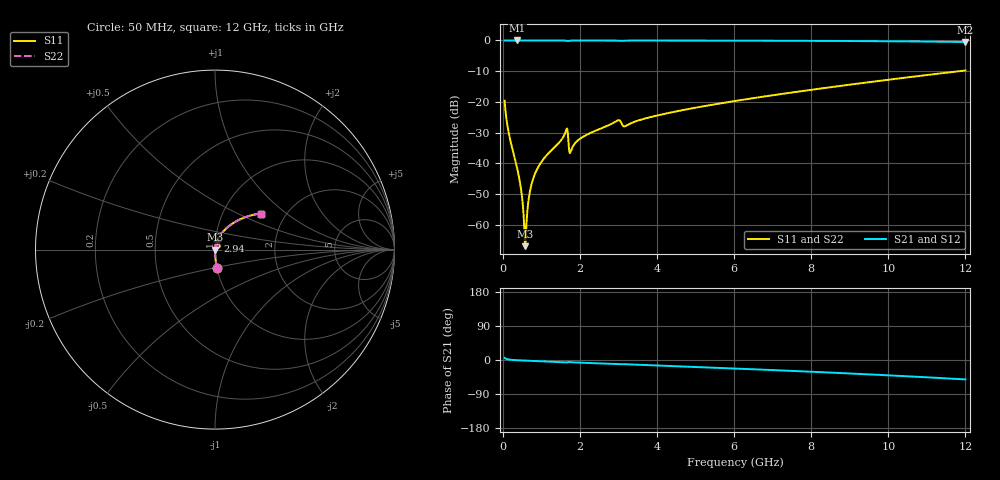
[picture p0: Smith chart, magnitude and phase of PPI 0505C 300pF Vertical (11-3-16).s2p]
# GHz S MA R 50
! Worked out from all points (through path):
!   1601 points, 50 MHz to 12 GHz, reference 50 ohm
!   highest |S21| = 0.00 dB at 378.6 MHz (marker M1); lowest = -0.5 dB at 12 GHz (marker M2)
!   group delay of S21, straight-line fit = 11.8 ps
!   lowest |S11| = -66.9 dB at 587.8 MHz (marker M3), VSWR 1.00, Z = 50 + j0.00658 ohm
!   |S11| at or under -10 dB: start of sweep to 11.84 GHz
!   |S22| runs from -66.9 to -9.8 dB; largest |S21 - S12| = 0
!   S11 on the Smith chart (normalised r, x): 50 MHz: 1.00, -0.21; 2.94 GHz: 1.02, +0.10; 12 GHz: 1.50, +0.68
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0.05  0.1046 -84.0  0.9943 5.9  0.9943 5.9  0.1046 -84.0
0.1769688  0.02721 -88.3  0.9993 1.1  0.9993 1.1  0.02721 -88.3
0.378625  0.008171 -87.9  0.9996 -0.6  0.9996 -0.6  0.008171 -87.9
0.4757188  0.00382 -84.9  0.9996 -1.1  0.9996 -1.1  0.00382 -84.9
0.5504062  0.0012 -70.3  0.9995 -1.5  0.9995 -1.5  0.0012 -70.3
0.58775  0.0004509 8.4  0.9995 -1.6  0.9995 -1.6  0.0004509 8.4
0.6250938  0.001288 67.5  0.9995 -1.8  0.9995 -1.8  0.001288 67.5
0.6848437  0.00293 78.7  0.9995 -2.1  0.9995 -2.1  0.00293 78.7
0.7520625  0.004682 81.6  0.9995 -2.4  0.9995 -2.4  0.004682 81.6
0.8491562  0.007051 83.0  0.9994 -2.8  0.9994 -2.8  0.007051 83.0
0.9835938  0.01013 83.6  0.9993 -3.3  0.9993 -3.3  0.01013 83.6
1.625906  0.03219 72.4  0.9931 -6.3  0.9931 -6.3  0.03219 72.4
1.655781  0.03633 60.9  0.9854 -6.5  0.9854 -6.5  0.03633 60.9
1.775281  0.0162 69.3  0.9956 -5.8  0.9956 -5.8  0.0162 69.3
2.044156  0.02615 80.5  0.9984 -7.2  0.9984 -7.2  0.02615 80.5
2.940406  0.04836 73.9  0.9942 -10.9  0.9942 -10.9  0.04836 73.9
3.179406  0.04027 70.0  0.9928 -11.1  0.9928 -11.1  0.04027 70.0
4.038312  0.06084 74.2  0.9967 -14.6  0.9967 -14.6  0.06084 74.2
6.025  0.1036 66.8  0.9929 -22.5  0.9929 -22.5  0.1036 66.8
8.019156  0.158 58.4  0.9853 -31.0  0.9853 -31.0  0.158 58.4
10.01331  0.2301 49.0  0.9705 -40.5  0.9705 -40.5  0.2301 49.0
12  0.3249 38.3  0.9424 -51.3  0.9424 -51.3  0.3249 38.3
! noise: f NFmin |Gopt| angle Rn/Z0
0.05  0.0003175  0.8363  0.2353  0.0004102
1.372  0.003378  0.6263  3.682  0.001691
2.701  0.006174  0.6037  7.172  0.002866
4.031  0.007251  0.523  10.37  0.002646
5.36  0.008586  0.4811  13.32  0.002788
6.682  0.01025  0.466  16.2  0.003183
8.012  0.01207  0.4615  18.99  0.003682
9.341  0.01408  0.4648  21.7  0.004301
10.67  0.01635  0.475  24.37  0.005084
12  0.01899  0.4915  27.04  0.006102
